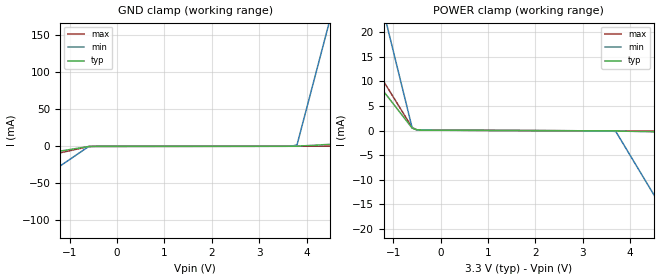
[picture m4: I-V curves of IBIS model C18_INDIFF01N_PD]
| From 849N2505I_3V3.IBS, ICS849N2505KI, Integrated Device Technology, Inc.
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[Model]   C18_INDIFF01N_PD
Model_type   Input
Polarity   Non-Inverting
Vinl = 0.8V
Vinh = 2.2V
|   typ   min   max
C_comp   2pF   1.5pF   2.5pF
|   typ   min   max
[Voltage range]   3.3V   3.135V   3.465V
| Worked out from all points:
|   GND clamp passes 1 mA (typ) near -0.67 V on its own axis
|   POWER clamp passes 1 mA (typ) near -0.64 V on its own axis
[GND_clamp]
|Voltage   I (typ)   I (min)   I (max)
-3.3V     -28.04mA   -118.2mA   -38.54mA
-600mV    -290.5uA   -393.5uA   -333.1uA
3.6V      78.06uA    99.07uA    79.3uA
3.8V      132.1uA    1.977mA    87.88uA
4.4V      2.329mA    148.1mA    142.9uA
4.5V      2.695mA    172.5mA    152uA
6.6V      10.38mA    683.9mA    344.5uA
[Power_clamp]
|Voltage   I (typ)   I (min)   I (max)
-3.3V     34.03mA    106.7mA    42.87mA
-2.3V     21.61mA    67.36mA    27.21mA
-2.2V     20.37mA    63.43mA    25.64mA
-2V       17.89mA    55.57mA    22.51mA
-1.9V     16.65mA    51.64mA    20.95mA
-1.2V     7.951mA    24.13mA    9.989mA
-1.1V     6.709mA    20.2mA     8.424mA
-600mV    498.2uA    551uA      596.3uA
-500mV    132.1uA    130.2uA    136.5uA
3.7V      -83.36uA   -211.1uA   -83.54uA
5V        -387.1uA   -21.08mA   -139.3uA
6.6V      -760.8uA   -46.77mA   -208uA
